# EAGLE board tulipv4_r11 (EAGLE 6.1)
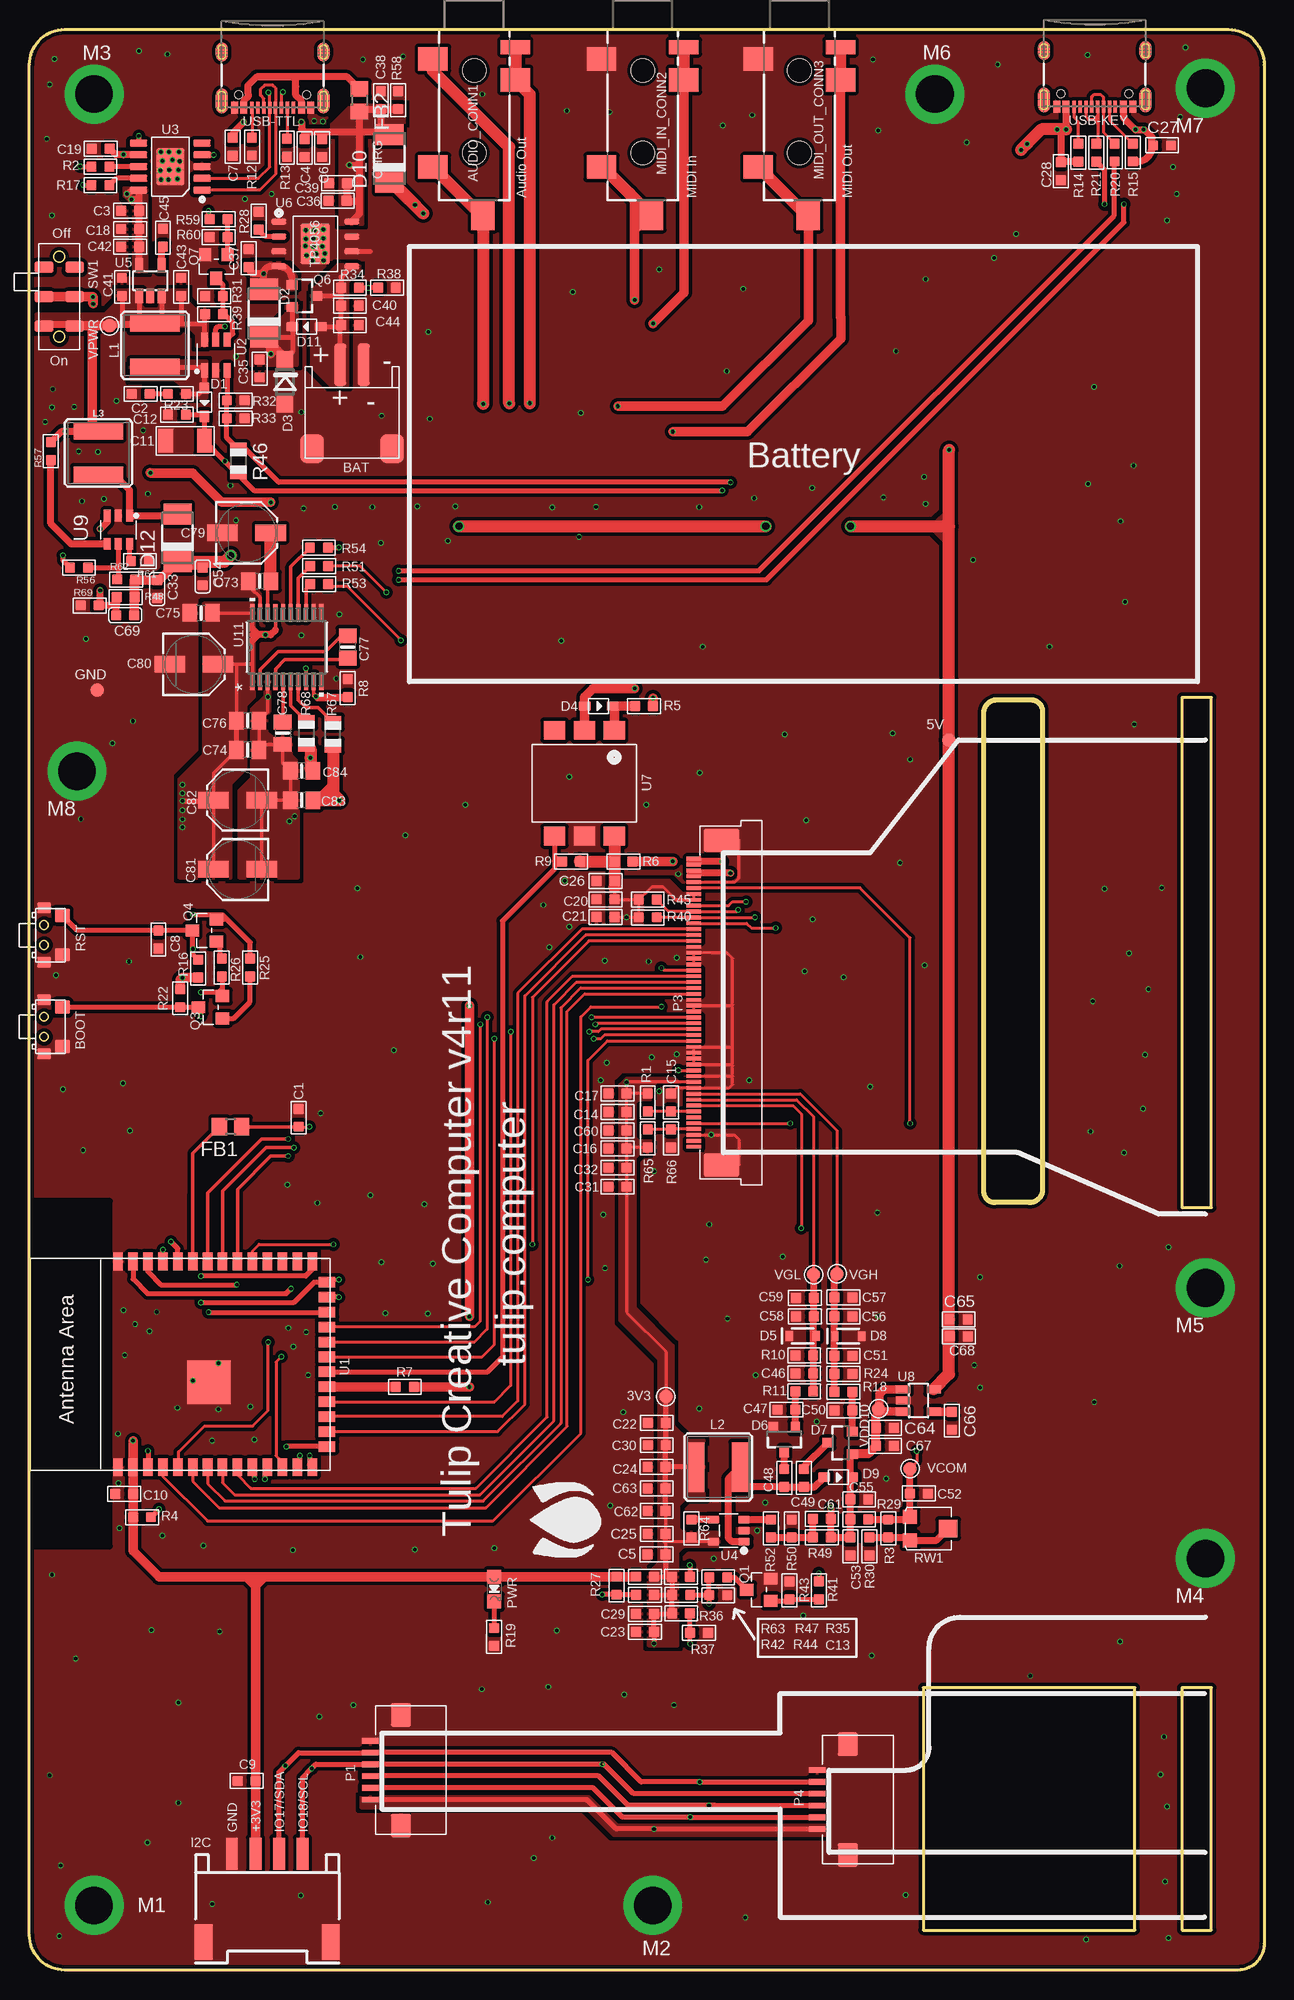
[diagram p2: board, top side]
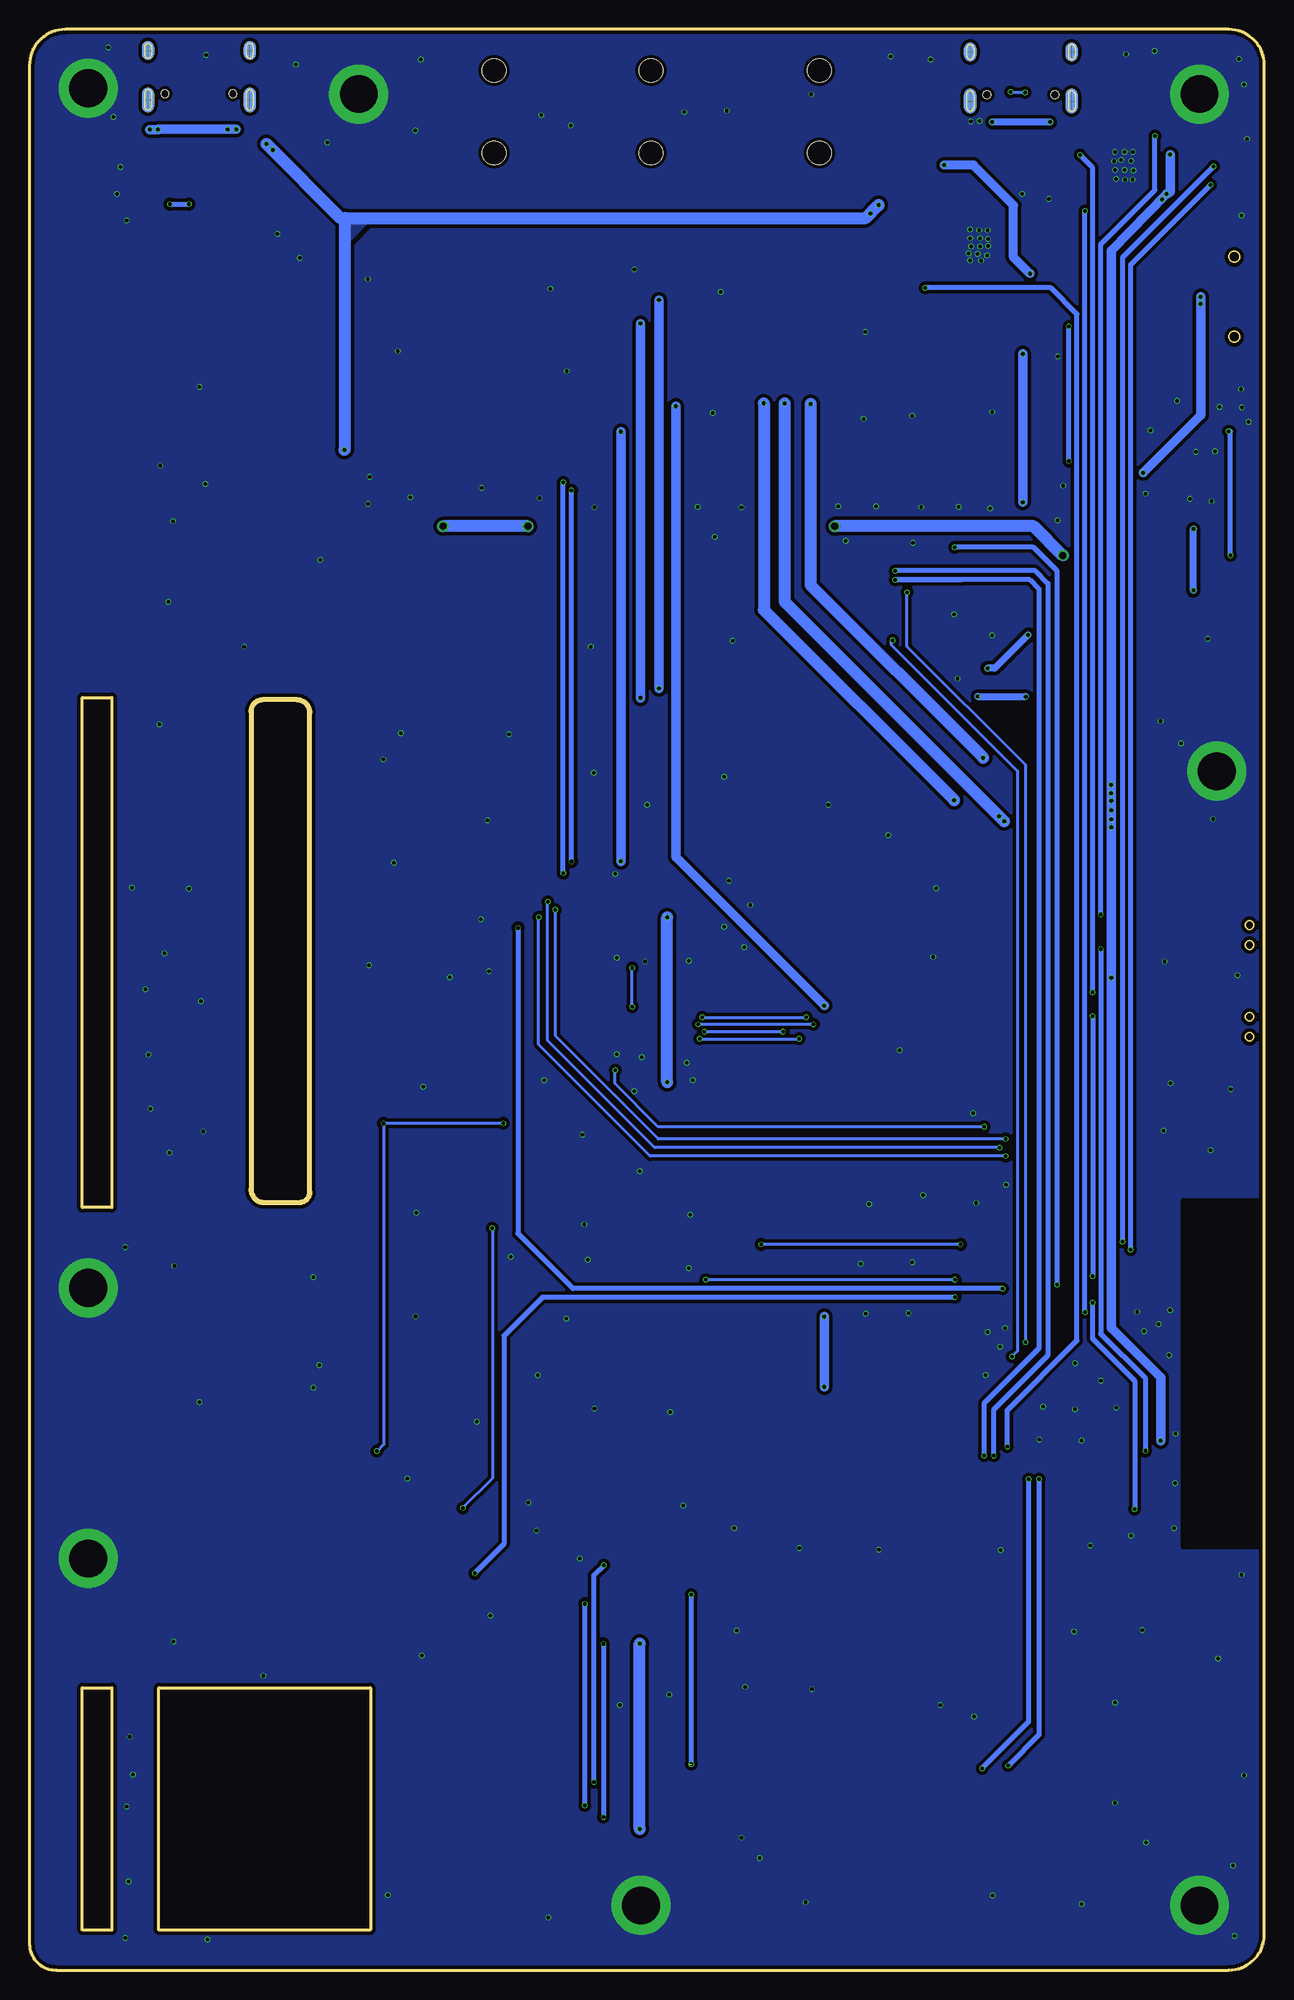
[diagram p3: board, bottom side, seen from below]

Size 105 x 165 mm. Coordinates in mm from the lower left corner, seen from the top.
Outline: 3,165 101.96,165 arc-90 105,161.96 105,2.26 arc-90 102.74,0 3,0 arc-90 0,3 0,162 arc-90 3,165
Outline: 85.03,65.25 82.09,65.25 arc-90 81.15,66.19 81.15,106.91 arc-90 82.25,108 85.17,108 arc-90 86.15,107.01 86.15,66.38 arc-90 85.03,65.25
Outline: 76,24 76,3.4 94,3.4 94,24 76,24
Outline: 98,108.2 98,64.82 100.5,64.82 100.5,108.2 98,108.2
Outline: 98,24 98,3.4 100.5,3.4 100.5,24 98,24
Copper layers (1*16): Top 0.035mm / dielectric 1.5mm / Bottom 0.035mm
Design rules: minimum track width 6mil, minimum drill 10mil, track to track 6mil, track to pad 6mil, pad to pad 6mil, via to via 6mil, smd to smd 0mil, copper to edge 10mil, drill to drill 10mil, minimum pad ring 3mil, minimum via ring 3mil, stop-mask expansion 2mil, vias tented up to drill 100mil, thermal gap 0mil
Net classes: 0 default: width 0.203 mm, drill 0.305 mm, clearance 0.152 mm; 1 vbat: width 0.254 mm, drill 0.305 mm, clearance 0.152 mm
tRestrict: area 0,36.1 to 6.8,65.4; area -3.4,136 to -2.6,142.5
bRestrict: area 0,36.1 to 6.8,65.4

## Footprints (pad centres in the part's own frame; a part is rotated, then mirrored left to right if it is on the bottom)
TP_4545 = smd 1.143 x 1.143: T 0,0
TP-D45MIL = smd 1.143 x 1.143: T 0,0
4UCONN_19269 = smd 2 x 2.5: 1 2.5,-3.5; 2 11.7,-3.5; 3 4.3,3.5 | smd 2.5 x 2: 4 15.8,0.75 | smd 1.2 x 2.5: 5 1.5,3.5 | hole 2: 3.5,0; 10.5,0
HW2-SMD-2.0-90D = smd 2 x 2.4: 3 3.4,-2.181; 4 -3.4,-2.181 | smd 1 x 3.6: + -1,4.953; - 1,4.953
2*4*3.5MM = smd 1.15 x 1.3: 1 -1.675,0; 2 1.675,0 | smd 0.9 x 1.2: 3 2.3,1.55; 4 -2.3,1.55
DISCRETE_C0603 = smd 0.889 x 0.889: 1 -0.762,0; 2 0.762,0
DISCRETE_C1206 = smd 1.27 x 2.032: 1 -1.651,0; 2 1.651,0
0603 = smd 0.889 x 0.889: 1 -0.762,0; 2 0.762,0
C0603 = smd 0.889 x 0.889: 1 0,0.762; 2 0,-0.762
0805-NO@1 = smd 1.24 x 1.5: 1 -0.95,0; 2 0.95,0
PANASONIC_C = smd 2.6 x 1.4: + 2.05,0; - -2.05,0
SOD323 = smd 1 x 0.8: + -1.2,0; - 1.2,0
DO-214AC = smd 1.8 x 2.4: A 2.025,0; C -2.025,0
SOD123 = smd 1.4 x 1.4: A 1.9,0; C -1.9,0
SOD-323 = smd 0.63 x 0.83: A 1.15,0; C -1.15,0
SOT23-3 = smd 0.8 x 0.9: 1 -0.95,-1; 2 0.95,-1; 3 0,1.1
R0805 = smd 1.3 x 1.5: 1 -0.95,0; 2 0.95,0
HW4-SMD-2.0-90D = smd 1.01 x 2.74: 1 -3,-0.1; 2 -1,-0.1; 3 1,-0.1; 4 3,-0.1 | smd 1.5 x 3: SS1 -5.4,7.4; SS2 5.4,7.4
CR54 = smd 4.2 x 1.4: P$1 0,1.85; P$2 0,-1.85
M2.5 = drill 3.2 pad 5: 1 0,0
1*6P-SMT1MM = smd 0.5 x 1.5: 1 -2.5,0; 2 -1.5,0; 3 -0.5,0; 4 0.5,0; 5 1.5,0; 6 2.5,0 | smd 2 x 1.7: 7 4.7,-2.6; 8 -4.7,-2.6
1*50P-SMT0.5MM = smd 0.3 x 1.3: 1 -12.25,0; 2 -11.75,0; 3 -11.25,0; 4 -10.75,0; 5 -10.25,0; 6 -9.75,0; 7 -9.25,0; 8 -8.75,0; 9 -8.25,0; 10 -7.75,0; 11 -7.25,0; 12 -6.75,0; 13 -6.25,0; 14 -5.75,0; 15 -5.25,0; 16 -4.75,0; 17 -4.25,0; 18 -3.75,0; 19 -3.25,0; 20 -2.75,0; 21 -2.25,0; 22 -1.75,0; 23 -1.25,0; 24 -0.75,0; 25 -0.25,0; 26 0.25,0; 27 0.75,0; 28 1.25,0; 29 1.75,0; 30 2.25,0; 31 2.75,0; 32 3.25,0; 33 3.75,0; 34 4.25,0; 35 4.75,0; 36 5.25,0; 37 5.75,0; 38 6.25,0; 39 6.75,0; 40 7.25,0; 41 7.75,0; 42 8.25,0; 43 8.75,0; 44 9.25,0; 45 9.75,0; 46 10.25,0; 47 10.75,0; 48 11.25,0; 49 11.75,0; 50 12.25,0 | smd 2 x 3: 51 13.79,-2.35; 52 -13.79,-2.35
CHIPLED_0805_NOOUTLINE = smd 1.2 x 1.2: A 0,-1.05; C 0,1.05
SOT23 = smd 1.016 x 1.143: 1 -0.95,-1.016; 2 0.95,-1.016; 3 0,1.016
DISCRETE_R0603 = smd 0.889 x 0.889: 1 -0.762,0; 2 0.762,0
R0603 = smd 0.889 x 0.889: 1 -0.762,0; 2 0.762,0
R0805' = smd 1.1 x 1.4: 1 -1,0; 2 1,0
TC33-3MM-SMD = smd 1.2 x 1.2: 1 -1,-1.625; 2 1,-1.625 | smd 1.5 x 1.6: 3 0,1.625
SMD-6-2.5MM = smd 1 x 1.6: 1 -2.5,1.3; 1@1 -2.5,-1.3; 2 0,1.3; 2@1 0,-1.3; 3 2.5,1.3; 3@1 2.5,-1.3
ESP32-­S2-­SOLO = smd 1.5 x 0.9: 1 -8.75,5.26; 2 -8.75,3.99; 3 -8.75,2.72; 4 -8.75,1.45; 5 -8.75,0.18; 6 -8.75,-1.09; 7 -8.75,-2.36; 8 -8.75,-3.63; 9 -8.75,-4.9; 10 -8.75,-6.17; 11 -8.75,-7.44; 12 -8.75,-8.71; 13 -8.75,-9.98; 14 -8.75,-11.25; 27 8.75,-11.25; 28 8.75,-9.98; 29 8.75,-8.71; 30 8.75,-7.44; 31 8.75,-6.17; 32 8.75,-4.9; 33 8.75,-3.63; 34 8.75,-2.36; 35 8.75,-1.09; 36 8.75,0.18; 37 8.75,1.45; 38 8.75,2.72; 39 8.75,3.99; 40 8.75,5.26 | smd 0.9 x 1.5: 15 -6.985,-12.5; 16 -5.715,-12.5; 17 -4.445,-12.5; 18 -3.175,-12.5; 19 -1.905,-12.5; 20 -0.635,-12.5; 21 0.635,-12.5; 22 1.905,-12.5; 23 3.175,-12.5; 24 4.445,-12.5; 25 5.715,-12.5; 26 6.985,-12.5 | smd 3.7 x 3.7: 41 -1.5,-2.46
SOT23-6 = smd 1.2 x 0.6: 1 -1.3,0.95; 2 -1.3,0; 3 -1.3,-0.95; 4 1.3,-0.95; 5 1.3,0; 6 1.3,0.95
ESOP-10-EP-150MIL = smd 1.5 x 0.6: 1 -2.7,2; 2 -2.7,1; 3 -2.7,0; 4 -2.7,-1; 5 -2.7,-2; 6 2.7,-2; 7 2.7,-1; 8 2.7,0; 9 2.7,1; 10 2.7,2 | smd 2.4 x 3.2: EP 0,0
SOT-23-5 = smd 0.7 x 1: 1 -0.95,-1.3; 2 0,-1.3; 3 0.95,-1.3; 4 0.95,1.3; 5 -0.95,1.3
SOT23-5 = smd 0.69 x 1.2: 1 -0.95,-1.3; 2 0,-1.3; 3 0.95,-1.3; 4 0.95,1.3; 5 -0.95,1.3
SOP8-1.27P = smd 1.27 x 0.51: 1 -3.1,1.905; 2 -3.1,0.635; 3 -3.1,-0.635; 4 -3.1,-1.905; 5 3.1,-1.905; 6 3.1,-0.635; 7 3.1,0.635; 8 3.1,1.905 | smd 2.5 x 3.4: 9 0,0
SOP-6-2.54MM = smd 1.6 x 1.8: 1 -4.5,2.54; 2 -4.5,0; 3 -4.5,-2.54; 4 4.5,-2.54; 5 4.5,0; 6 4.5,2.54
SOT-23-6 = smd 1 x 0.6: 1 -1.2,0.95; 2 -1.2,0; 3 -1.2,-0.95; 4 1.2,-0.95; 5 1.2,0; 6 1.2,0.95
PW20_TEX = smd 1.473 x 0.356: 1 -2.921,2.925; 2 -2.921,2.275; 3 -2.921,1.625; 4 -2.921,0.975; 5 -2.921,0.325; 6 -2.921,-0.325; 7 -2.921,-0.975; 8 -2.921,-1.625; 9 -2.921,-2.275; 10 -2.921,-2.925; 11 2.921,-2.925; 12 2.921,-2.275; 13 2.921,-1.625; 14 2.921,-0.975; 15 2.921,-0.325; 16 2.921,0.325; 17 2.921,0.975; 18 2.921,1.625; 19 2.921,2.275; 20 2.921,2.925
USB-C-16P-5 = smd 0.3 x 1: A5 -1.25,-0.34; A6 -0.25,-0.34; A7 0.25,-0.34; A8 1.25,-0.34; B5 1.75,-0.34; B6 0.75,-0.34; B7 -0.75,-0.34; B8 -1.75,-0.34 | smd 0.6 x 1: GND -3.225,-0.34; GND2 3.225,-0.34; VBUS1 -2.45,-0.34; VBUS2 2.45,-0.34 | smd 1 x 2.1: SHLD1 -4.32,-0.915; SHLD2 4.32,-0.915 | smd 1 x 2.1 bottom: SHLD3 -4.32,-0.915; SHLD4 4.32,-0.915 | smd 1 x 1.6: SHLD5 -4.32,-5.095; SHLD8 4.32,-5.095 | smd 1 x 1.6 bottom: SHLD6 -4.32,-5.095; SHLD7 4.32,-5.095 | hole 0.65: -2.89,-1.445; 2.89,-1.445

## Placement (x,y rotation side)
3V3  [TP_4545]  54.13,48.77 270 top
5V  [TP-D45MIL]  78.18,104.57 0 top
AUDIO_CONN1  19269  [4UCONN_19269]  37.82,165 270 top
BAT  JST-2P  [HW2-SMD-2.0-90D]  27.43,131.53 0 top
BOOT  TS24CA  [2*4*3.5MM]  2.8,80.2 90 top
C1  10pF/25V  [DISCRETE_C0603]  22.89,72.47 270 top
C2  10pF/50V  [DISCRETE_C0603]  9.47,134.01 0 top
C3  10uF  [DISCRETE_C0603]  8.56,149.58 0 top
C4  10uF  [DISCRETE_C0603]  23.39,154.91 90 top
C5  10uF  [DISCRETE_C0603]  53.31,35.36 0 top
C6  10uF  [DISCRETE_C0603]  24.89,154.91 90 top
C7  0.1uF  [DISCRETE_C0603]  17.3,155.02 90 top
C8  0.1uF  [DISCRETE_C0603]  10.97,87.63 270 top
C9  0.1uF  [DISCRETE_C0603]  18.47,16.08 180 top
C10  10uF  [DISCRETE_C0603]  8.05,40.49 180 top
C11  4.7uF/35V  [DISCRETE_C1206]  13.23,130.02 0 top
C12  0.1uF/50V  [DISCRETE_C0603]  12.55,132.23 0 top
C13  NC  [DISCRETE_C0603]  58.57,31.88 180 top
C14  0.1uF  [DISCRETE_C0603]  50.01,72.95 180 top
C15  100nF  [DISCRETE_C0603]  54.56,73.76 270 top
C16  10uF  [DISCRETE_C0603]  50.01,69.85 0 top
C17  0.1uF  [DISCRETE_C0603]  50.01,74.52 0 top
C18  0.1uF  [DISCRETE_C0603]  8.56,148.03 0 top
C19  0.1uF  [DISCRETE_C0603]  6.07,154.86 0 top
C20  10uF  [DISCRETE_C0603]  48.99,91.04 0 top
C21  0.1uF  [DISCRETE_C0603]  49,89.54 0 top
C22  10uF  [0603]  53.35,46.52 180 top
C23  10uF  [DISCRETE_C0603]  52.34,28.76 0 top
C24  0.1uF  [DISCRETE_C0603]  53.34,42.77 0 top
C25  0.1uF  [DISCRETE_C0603]  53.34,37.08 0 top
C26  0.1uF  [DISCRETE_C0603]  49,92.58 0 top
C27  10uF  [0603]  96.31,155.14 0 top
C28  0.1uF  [DISCRETE_C0603]  87.71,152.95 90 top
C29  10uF  [DISCRETE_C0603]  52.35,30.3 0 top
C30  0.1uF  [DISCRETE_C0603]  53.35,44.63 0 top
C31  10uF  [DISCRETE_C0603]  50.01,66.61 180 top
C32  0.1uF  [DISCRETE_C0603]  50.01,68.22 180 top
C33  22uF  [C0603]  10.87,117.42 0 top
C35  10uF  [0603]  19.58,136.17 90 top
C36  10uF  [0603]  26.21,150.44 0 top
C37  0.1uF  [0603]  18.63,145.55 90 top
C38  10uF  [0603]  29.88,158.99 90 top
C39  0.1uF  [0603]  26.25,151.93 180 top
C40  10uF  [0603]  27.25,141.5 0 top
C41  4.7uF/16V  [0603]  7.87,143.1 90 top
C42  10uF  [0603]  8.56,146.53 180 top
C43  10uF  [0603]  12.9,143.1 270 top
C44  0.1uF  [0603]  27.25,139.85 0 top
C45  NC  [0603]  11.35,147.29 90 top
C46  0.1uF  [DISCRETE_C0603]  65.89,50.72 0 top
C47  0.1uF  [DISCRETE_C0603]  64.36,47.65 0 top
C48  0.1uF  [DISCRETE_C0603]  64.19,41.83 90 top
C49  0.1uF  [DISCRETE_C0603]  65.86,41.83 270 top
C50  0.1uF  [DISCRETE_C0603]  69.22,47.57 0 top
C51  0.1uF  [DISCRETE_C0603]  69.22,52.22 180 top
C52  0.1uF  [DISCRETE_C0603]  75.64,40.51 180 top
C53  0.1uF  [DISCRETE_C0603]  69.8,36.02 90 top
C54  100nF  [C0603]  14.73,118.49 0 top
C55  0.1uF  [DISCRETE_C0603]  70.56,40.03 180 top
C56  1uF  [DISCRETE_C0603]  69.22,55.58 180 top
C57  1uF  [DISCRETE_C0603]  69.22,57.2 180 top
C58  1uF  [DISCRETE_C0603]  65.94,55.58 0 top
C59  1uF  [DISCRETE_C0603]  65.94,57.15 0 top
C60  100nF  [DISCRETE_C0603]  50.01,71.37 0 top
C61  10pF/25V  [DISCRETE_C0603]  67.39,38.35 0 top
C62  0.1uF  [DISCRETE_C0603]  53.34,39.04 0 top
C63  10uF  [DISCRETE_C0603]  53.34,40.97 0 top
C64  4.7uF/16V  [0603]  72.76,44.57 0 top
C65  10uF  [0603]  79.01,55.32 0 top
C66  NC  [0603]  78.46,46.71 270 top
C67  0.1uF/16V  [DISCRETE_C0603]  72.76,46.1 180 top
C68  0.1uF  [DISCRETE_C0603]  79.03,53.87 180 top
C69  22pF  [C0603]  8.15,115.19 270 top
C73  0.1uF  [0805-NO@1]  19.58,118.08 180 top
C74  0.1uF  [0805-NO@1]  18.57,103.73 180 top
C75  0.1uF  [0805-NO@1]  14.6,115.39 0 top
C76  0.1uF  [0805-NO@1]  18.57,106.22 180 top
C77  2.2uF  [0805-NO@1]  27.08,112.5 90 top
C78  2.2uF  [0805-NO@1]  21.54,105.16 270 top
C79  10uF  [PANASONIC_C]  18.47,122.2 0 top
C80  10uF  [PANASONIC_C]  14,111.02 0 top
C81  10uF  [PANASONIC_C]  17.7,93.57 180 top
C82  10uF  [PANASONIC_C]  17.7,99.47 180 top
C83  2.2nF  [0805-NO@1]  23.16,99.47 180 top
C84  2.2nF  [0805-NO@1]  23.16,101.96 180 top
D1  1N4148WS  [SOD323]  14.88,133.3 270 top
D2  SS54  [DO-214AC]  19.96,140.87 90 top
D3  W8/5.1V  [SOD123]  21.72,135.03 270 top
D4  1N4148WS  [SOD323]  48.41,107.47 0 top
D5  7.5V  [SOD-323]  65.76,53.92 0 top
D6  200mA/70V  [SOT23-3]  64.19,45.16 180 top
D7  200mA/70V  [SOT23-3]  68.99,44.83 90 top
D8  16V  [SOD-323]  69.62,53.9 0 top
D9  1N4148WS  [SOD323]  68.78,41.91 0 top
D10  SS54  [DO-214AC]  30.62,154.02 90 top
D11  B5819WS  [SOD323]  23.57,139.73 180 top
D12  SS54  [DO-214AC]  12.6,121.77 90 top
FB1  100Mhz@120R  [R0805]  17.1,71.7 180 top
FB2  100Mhz@120R  [R0805]  28.06,158.98 270 top
GND  [TP-D45MIL]  5.77,108.81 0 top
I2C  [HW4-SMD-2.0-90D]  20.22,9.79 180 top
L1  10µH/±30%  [CR54]  10.67,138.15 0 top
L2  10µH/±30%  [CR54]  58.57,42.77 90 top
L3  3.3µH/±30%/3.4A  [CR54]  5.87,128.98 0 top
M1  M2.5  [M2.5]  5.5,5.5 0 top
M2  M2.5  [M2.5]  53,5.5 0 top
M3  M2.5  [M2.5]  5.5,159.5 0 top
M4  M2.5  [M2.5]  100,35 0 top
M5  M2.5  [M2.5]  100,58 0 top
M6  M2.5  [M2.5]  77,159.5 0 top
M7  M2.5  [M2.5]  100,160 0 top
M8  M2.5  [M2.5]  4.04,101.93 0 top
MIDI_IN_CONN2  19269  [4UCONN_19269]  52.15,165 270 top
MIDI_OUT_CONN3  19269  [4UCONN_19269]  65.48,165 270 top
P1  1X6P-1MM  [1*6P-SMT1MM]  29,17 90 top
P3  150P-0.5MM  [1*50P-SMT0.5MM]  56.5,82.25 90 top
P4  1X6P-1MM  [1*6P-SMT1MM]  67,14.5 90 top
PWR  NC  [CHIPLED_0805_NOOUTLINE]  39.52,32.4 180 top
Q1  S8050  [SOT23]  62.03,32.33 90 top
Q3  S8050  [SOT23]  15.41,81.86 90 top
Q4  S8050  [SOT23]  14.88,88.39 90 top
Q6  MOSFET-PCHANNEL  [SOT23-3]  23.34,142.34 270 top
Q7  S8050  [SOT23]  15.9,144.83 180 top
R1  10K  [DISCRETE_R0603]  52.58,73.76 90 top
R2  0R  [R0603]  6.05,153.34 0 top
R3  3.48K  [DISCRETE_R0603]  73.03,37.54 90 top
R4  NC  [R0603]  9.58,38.51 0 top
R5  220R  [R0603]  52.27,107.47 0 top
R6  33R  [R0603]  50.52,94.26 0 top
R7  10R  [R0603]  31.93,49.58 0 top
R8  0R  [DISCRETE_R0603]  27.08,108.99 90 top
R9  470R  [R0603]  46.05,94.26 180 top
R10  4.3K  [DISCRETE_R0603]  65.89,52.27 0 top
R11  2K  [DISCRETE_R0603]  65.89,49.2 0 top
R12  5.1K  [DISCRETE_R0603]  18.92,155.04 90 top
R13  5.1K  [DISCRETE_R0603]  21.89,154.94 90 top
R14  56K  [DISCRETE_R0603]  89.2,154.51 90 top
R15  56K  [DISCRETE_R0603]  93.83,154.53 90 top
R16  10K  [R0603]  14.35,85.14 270 top
R17  0R  [R0603]  6.05,151.76 0 top
R18  1.2K  [DISCRETE_R0603]  69.22,49.15 0 top
R19  NC  [DISCRETE_R0603]  39.52,28.32 90 top
R20  51R  [R0603]  92.28,154.53 270 top
R21  51R  [R0603]  90.73,154.51 270 top
R22  10K  [R0603]  12.83,82.63 90 top
R23  50R  [DISCRETE_R0603]  12.55,134.01 0 top
R24  4.3K  [DISCRETE_R0603]  69.22,50.7 180 top
R25  10K  [R0603]  18.77,85.24 90 top
R26  10K  [R0603]  16.37,85.24 270 top
R27  NC  [R0603]  49.91,32.69 90 top
R28  1.2K  [R0603]  19.48,148.74 90 top
R29  10KR  [DISCRETE_R0603]  70.56,38.33 180 top
R30  2K  [DISCRETE_R0603]  71.42,36.02 90 top
R31  NC  [DISCRETE_R0603]  15.7,142.32 0 top
R32  3.6R  [DISCRETE_R0603]  17.55,133.45 180 top
R33  3.6R  [DISCRETE_R0603]  17.55,131.93 180 top
R34  470K  [R0603]  27.25,143.03 180 top
R35  0R  [R0603]  58.57,33.4 180 top
R36  NC  [DISCRETE_R0603]  55.42,30.33 180 top
R37  NC  [DISCRETE_R0603]  56.95,28.68 0 top
R38  470K  [R0603]  30.4,143.03 180 top
R39  10K  [DISCRETE_R0603]  15.7,140.79 180 top
R40  10K  [DISCRETE_R0603]  52.58,89.51 180 top
R41  4.7K  [DISCRETE_R0603]  67.13,32.28 90 top
R42  5.1K  [DISCRETE_R0603]  52.35,31.91 0 top
R43  10K  [DISCRETE_R0603]  64.64,32.28 270 top
R44  10K  [DISCRETE_R0603]  55.43,31.9 180 top
R45  10K  [DISCRETE_R0603]  52.58,91.01 180 top
R46  470  [R0805']  17.79,128.31 90 top
R47  5.1K  [DISCRETE_R0603]  55.41,33.43 180 top
R48  88.7K  [DISCRETE_R0603]  8.18,116.74 0 top
R49  100K  [DISCRETE_R0603]  67.39,36.78 0 top
R50  13K  [DISCRETE_R0603]  64.82,37.54 270 top
R51  0R  [R0603]  24.64,119.35 180 top
R52  100K  [DISCRETE_R0603]  63.07,37.54 90 top
R53  0R  [R0603]  24.64,117.83 180 top
R54  0R  [R0603]  24.61,120.95 180 top
R56  NC  [DISCRETE_R0603]  4.22,119.25 180 top
R57  100K  [DISCRETE_R0603]  1.83,129.13 90 top
R58  100k  [R0603]  31.34,158.99 90 top
R59  4.7K  [DISCRETE_R0603]  16.1,148.87 180 top
R60  10K  [DISCRETE_R0603]  16.1,147.35 0 top
R61  NC  [DISCRETE_R0603]  9.4,119.79 180 top
R62  0R  [DISCRETE_R0603]  8.23,118.24 0 top
R63  0R  [R0603]  52.35,33.45 0 top
R64  4.3K  [DISCRETE_R0603]  56.29,37.54 270 top
R65  10K  [DISCRETE_R0603]  52.58,70.71 270 top
R66  NC  [DISCRETE_R0603]  54.56,70.71 90 top
R67  470  [R0805']  25.81,105.08 90 top
R68  470  [R0805']  23.57,105.16 90 top
R69  12K  [DISCRETE_R0603]  5.13,116.03 0 top
RST  TS24CA  [2*4*3.5MM]  2.8,88 90 top
RW1  TC33X-2-103E  [TC33-3MM-SMD]  76.5,37.54 270 top
SW1  JS102011JAQN  [SMD-6-2.5MM]  2.54,142.27 270 top
U1  ESP32­S2­SOLO  [ESP32-­S2-­SOLO]  12.8,51.5 90 top
U2  RY3730  [SOT23-6]  15.85,137.31 90 top
U3  CH340K  [ESOP-10-EP-150MIL]  11.99,153.34 180 top
U4  SGM6601YTN5G/TR  [SOT-23-5]  59.46,37.36 90 top
U5  SPX3819  [SOT23-5]  10.29,143.64 0 top
U6  TP4056  [SOP8-1.27P]  24.31,146.76 0 top
U7  H11L1SR2M  [SOP-6-2.54MM]  47.19,100.91 270 top
U8  SPX3819  [SOT23-5]  75.6,48.43 270 top
U9  HX3608  [SOT-23-6]  7.57,122.45 270 top
U11  U11  [PW20_TEX]  21.89,112.47 90 top
USB-KEY  [USB-C-16P-5]  90.58,158.1 180 top
USB-TTL  [USB-C-16P-5]  20.69,157.99 180 top
VCOM  [TP_4545]  74.88,42.62 0 top
VDD10  [TP_4545]  72.21,47.72 0 top
VGH  [TP_4545]  68.68,59.21 0 top
VGL  [TP_4545]  66.67,59.13 90 top
VPWR  [TP_4545]  6.81,139.8 0 top

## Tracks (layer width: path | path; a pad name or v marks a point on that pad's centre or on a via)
3.3V  (via drill 0.3)
  Top 0.254: C16.2 C60.2 C14.1 C17.2 | R65.2 50.77,69.95 C16.2 | R1.2 C17.2 | C17.2 v50.77,75.5 P3.12 | R45.2 52.91,92.1 53.9,92.1 55,91 P3.43 P3.44 | R45.2 R40.2 51.79,89.54 C21.2 | C20.2 51.79,91.04 R45.2 | C16.2 C32.1 C31.1 50.78,55.93 54.11,52.59 C22.1 54.08,46.49 54.08,36.41 | 54.08,36.41 C5.2 | U4.5 56.31,36.41 | 56.31,36.41 54.08,36.41 | R64.2 56.31,36.78 56.31,36.41 | R6.1 49.76,95.68 49.73,95.71
  Top 0.305: C20.2 49.76,92.05 C26.2
  Top 0.406: P4.1 v53.11,12 49.9,12 47.4,14.5 P1.1 | R44.2 R36.2 54.63,30.3 C29.2 C23.2 v53.11,27.77 v53.11,27.76 | R42.2 54.65,31.91 R44.2 | R44.2 54.66,33.41 R47.2 54.62,33.45 54.05,33.45 | R63.2 54.05,33.45 | C5.2 54.08,33.48 54.05,33.45 | L2.P$1 C24.2 | 54.08,36.41 54.08,37.06 C25.2 | C62.2 C63.2 C24.2 | C24.2 C30.2 C22.1 54.11,48.75 3V3.T
  Top 1.016: R9.1 R6.1 | U7.6 49.73,95.71 49.73,92.07 49.76,92.05
  Bottom 1.016: v50.77,75.5 v50.77,89.5 | v53.11,12 v53.11,27.76
  pour Top: 28.22,14.76 47.6,14.76 50.01,12.34 67.74,12.34 67.74,11.43 49.68,11.43 47.35,13.77 28.22,13.77
  pour Top: 52.65,27.53 52.65,33.78 53.54,34.67 53.54,51.87 50.22,55.19 50.22,75.31 50.77,75.87 54.71,75.87 55.35,75.46 55.32,75.46 53.26,75.41 52.88,75.03 52.88,73.99 51.79,73.99 51.49,73.69 51.49,70.84 51.79,70.54 52.86,70.54 52.86,69.44 51.92,69.44 51.49,69.01 51.49,56.36 54.74,53.11 54.74,46.35 56.03,45.06 57.38,45.06 57.38,40.08 55.8,40.08 55.19,39.47 55.19,37.59 55.52,37.26 58.62,37.26 58.62,35.97 55.63,35.97 55.12,35.46 55.12,27.53
  pour Top: 49.35,89 52.2,89 52.2,91.29 52.78,91.87 53.98,91.87 54.89,90.96 57,90.96 57,91.54 55.58,91.54 54.48,92.63 50.04,92.63 49.35,91.95
5V  (via drill 0.3, 0.6)
  Top 0.254: 33.5,149.34 v33.48,149.34 arc-90 v33.48,149.35 | v33.48,149.35 arc90 v33.48,149.35
  Top 0.406: C28.2 87.72,153.73 87.72,153.74 | D10.C 30.59,152 30.59,151.84
  Top 0.584: v88.13,156.5 v88.14,156.5 | v88.14,156.5 arc90 v88.14,156.5
  Top 0.61: USB-KEY.VBUS1 93.03,157.49 94.06,156.46 94.11,156.46 | USB-KEY.VBUS2 88.13,157.08 v88.14,156.5 | 94.11,156.46 94.82,156.46 95.38,155.91 arc-90 95.38,155.9 95.38,155.88 arc-90 95.45,155.81 95.45,155.68 | v94.06,156.49 94.08,156.49 94.11,156.46 | R15.1 94.22,153.77 arc90 95.45,155 95.45,155.68 | R14.1 87.7,153.75 arc90 87.69,153.74 87.72,153.74 arc90 87.74,153.76 87.74,156.11 arc-90 v88.13,156.5 | C27.1 95.45,155.68 | 8.94,118.19 C33.1 10.87,118.16 10.95,118.16 12.17,119.38 14.61,119.38 C54.1 | 5V.T 78.23,104.57 78.23,104.64 78.2,104.67
  Top 0.711: 78.25,53.87 C68.2 78.25,53.87 | 78.25,53.87 78.21,53.91 78.16,53.91 78.09,53.84 | 78.25,53.87 78.2,53.83 | C65.1 78.2,55.28
  Top 0.813: C69.1 8.91,118.16 | 8.91,118.16 8.94,118.19 | 8.91,118.16 10.87,118.16 11.02,118.16 D12.C | R48.2 8.94,118.19 | 8.94,118.19 R62.2
  Top 1.016: v88.14,156.5 86.07,156.5 v84.84,155.27 v84.32,154.75 v84.31,154.75 | v32.8,150.08 31.04,151.84 31.01,151.84 | 31.01,151.84 30.59,151.84 30.28,151.84 | 30.46,151.65 31.2,151.65 | 31.2,151.65 33.5,149.34 | 31.2,151.65 31.01,151.84 | U8.5 78.2,50.68 78.2,53.83 78.2,55.28 78.2,104.67 78.2,122.73 | 78.2,122.73 v78.2,129.26 | D12.C 16.59,119.74 v17.12,120.27 | v36.52,122.76 v62.61,122.76 | v69.83,122.76 78.03,122.76 arc-90 78.05,122.73 78.2,122.73
  Bottom 0.584: v87.4,156.5 arc90 v87.39,156.49 | v94.06,156.48 arc-90 v94.06,156.49
  Bottom 0.61: 94.05,156.5 v94.06,156.49
  Bottom 0.813: 94.05,156.5 v88.14,156.5 v87.4,156.5 | v94.76,156.48 v94.06,156.48
  Bottom 1.016: 78.53,148.96 v84.84,155.27 | 78.53,148.96 78.16,148.96 | 78.16,148.96 33.88,148.96 32.8,150.04 v32.8,150.08 | v78.2,129.26 78.16,129.3 78.16,148.96 | 78.53,148.96 78.49,148.93 78.05,148.93 78.08,148.96 78.14,148.96 78.14,148.91 | v17.12,120.27 19.61,122.76 v36.52,122.76 | v62.61,122.76 v69.83,122.76
  pour Bottom: 75.98,148.82 77.87,146.93 78.54,146.93 78.43,147.59 78.49,149.27 75.98,149.27
  pour Top: 78,124.1 76.83,122.94 76.83,122.38 77.83,121.39 78.05,121.39 78.05,124.13 78.03,124.13
+3V3  (via drill 0.3)
  Top 0.305: 18.97,113.56 U11.20 C75.2 | 18.97,113.56 18.97,110.9 | U11.1 | U11.17 20.92,113.94 | 19,113.54 18.97,113.56 | C80.+ 17.7,111.02 | 17.7,111.02 18.84,111.02 18.97,110.9 | C76.2 17.62,110.94 17.7,111.02 | C74.2 15.65,101.77 C82.+ C81.+ | U11.8 v23.52,110.69 | v23.52,110.69 | U11.1 18.97,110.9 | 18.97,110.9
  Top 0.406: 8.02,154.34 v8,154.36 | C74.2 C76.2 | v13,99.4 15.59,99.4 C82.+
  Top 0.61: 20.92,113.94 20.52,113.54 v20.06,113.54 19.43,113.54 | 19.43,113.54 19,113.54 | U3.7 8.02,154.34 7.36,154.34 C19.2 | v8.31,151 8.74,151.34 U3.10 9.32,151.31 9.32,150.44 | 18.85,114.22 18.85,114.12 19.43,113.54 | 19.43,113.54 18.82,112.93 | U5.5 9.34,146.52 C42.1 C18.2 C3.2 9.32,150.44 | v8.69,150.55 9.22,150.55 9.32,150.44
  Top 0.813: 19.48,33.45 11.04,33.45 11.02,33.43 8.81,35.64 R4.1 C10.1 U1.2 v8.81,45 | 19.48,33.45 PWR.A R27.2 R63.1 | I2C.3 C9.1 19.23,32.69 | 19.23,32.69 19.23,33.19 19.48,33.45 | R22.2 12.83,84.21 v13,84.38 R16.2 | 19.23,32.69 19.99,33.45 | 19.23,32.69 19.18,32.69 18.47,33.4
  Bottom 0.61: v20.06,113.54 22.91,110.69 v23.52,110.69
  Bottom 0.813: v8.81,45 8.81,50.39 13,54.58 v13,84.38 v13,99.4 13,146.21 v8.31,151 8,151.21 v8,154.36
  other vias: 13.03,100.77 13,97.83 13.03,100.06 13,98.61 13,97.16
  pour Top: 15.44,116.26 19.1,116.26 19.1,108.18 18.39,107.47 18.39,102.08 17.12,100.81 17.12,92.81 12.75,92.81 12.75,101.3 14.83,103.38 14.83,116.26
  pour Top: 8.86,144.35 8.86,149.99 8.05,150.8 8.05,151.56 9.96,151.56 9.96,144.4 9.96,144.35
AGND  (via drill 0.3)  (1 unrouted)
  Top 0.254: R8.1 24.49,108.23 24.17,108.55 U11.9 24.17,108.29 v24.35,108.28
  Top 0.305: C81.- C82.- C83.2 C84.2 21.54,102.63 C78.2 19.63,104.21 19.52,104.32 | C74.1 19.52,104.32 | 19.52,104.32 C76.1 20.27,106.97 v20.27,108.25 U11.3 | 24.18,108.84 24.18,108.31 24.49,108 27.15,108 27.15,108.43 27.03,108.43 26.95,108.36 24.41,108.36 24.23,108.53
  Top 0.406: AUDIO_CONN1.1 34.32,161.97
  Top 1.016: v40.79,133.2 40.79,154.99 34.32,161.46 AUDIO_CONN1.1
  Bottom 0.254: 20.3,108.28 v20.27,108.25
  Bottom 0.61: v24.35,108.28 20.3,108.28
  Bottom 1.016: v40.79,133.2 40.79,116.36 v22.1,97.66
  other vias: 22.56,98.09
  pour Top: 17.86,92.81 17.86,100.33 18.9,101.37 18.9,107.24 20.04,108.38 20.04,110.29 20.42,110.29 20.42,106.96 20.19,106.73 20.19,105.31 20.6,104.9 22.28,104.9 22.28,103.33 22.83,102.77 22.83,92.89 22.83,92.81
AVDD10  (via drill 0.3)
  Top 0.254: P3.8 64.93,73.5 65.63,72.8 v65.63,63.07
  Top 0.61: v68.15,39.29 C61.2 R49.2 C53.2 R29.2 C55.2 69.8,41.96 | 69.8,41.96 69.8,43.69 D7.1 | D9.- 69.85,41.91 69.8,41.96
  Top 0.711: U8.3 72.42,47.48 72.29,47.61 72.29,47.78 | U8.1 72.66,49.38 72.29,49 72.29,47.78 | VDD10.T 72.21,47.78 72.18,47.81 72.27,47.81 72.29,47.78
  Top 0.762: C64.1 71.32,43.89 70,43.89 D7.1 | C64.1 | C64.1 C67.2 72,47.06 72.42,47.48
  Bottom 0.254: v65.63,63.07 65.63,41.81 v68.15,39.29
BCLK
  Top 0.305: U11.13 23.52,117.47 R53.2
D+
  Top 0.254: U3.1 19.58,151.33 20.94,152.69 USB-TTL.A6 20.94,160.04 20.7,160.27 19.99,160.27 19.66,159.94 19.66,159.38 19.94,159.11 USB-TTL.B6
D-  (via drill 0.3)
  Top 0.254: U3.2 19.47,152.34 20.44,153.31 USB-TTL.A7 20.44,159.52 v20.32,159.64 | USB-TTL.B7 21.44,159.54 v21.57,159.66
  Bottom 0.254: v21.57,159.66 v20.32,159.64
DCLK  (via drill 0.3)
  Top 0.254: C1.2 v23.8,71.7 | 56.33,76.5 P3.14 v55.2,76.5 v55.19,76.5
  Top 0.305: FB1.1 | FB1.1 C1.2
  Bottom 0.254: v23.8,71.7 51.54,71.7 55.19,75.36 v55.19,76.5
DIN
  Top 0.305: U11.14 22.87,118.35 R51.2
DTR  (via drill 0.3)
  Top 0.406: U3.4 v15.66,154.34 v15.67,154.33 | Q3.2 16.42,83.44 | 16.42,83.44 16.42,84.42 R26.2 | v14.58,83.14 16.13,83.14 16.42,83.44
  Bottom 0.406: v14.58,83.14 14.58,153.24 v15.67,154.33
ENABLE
  Top 0.61: U9.4 3.56,121.26 1.83,122.99 R57.1
GND  (via drill 0.3)
  Top 0.254: P3.51 60.35,96.04 60.35,92.86 59.99,92.5 P3.46 | v57.96,71.02 56.14,71 P3.3 59.96,71 60.35,70.61 60.35,68.46 P3.52 | 59.79,76 59.79,75.29 59.51,75 P3.11 55.04,75 C15.1 | 59.79,76 59.79,76.91 | 59.79,76.91 59.79,82.07 | 59.79,82.07 59.79,86.03 59.33,86.49 58.01,86.49 P3.34 P3.32 | P3.13 59.79,76 | 59.79,76.91 59.7,77 P3.15 P3.18 59.73,78.5 59.74,78.51 | 59.79,82.07 59.72,82 P3.25 P3.24
  Top 0.305: U11.19 19.62,116.73 18.87,117.47 18.87,117.85 C73.2
  Top 0.406: U6.6 29.01,146.13
  other vias: 96.47,19.84 96.57,7.54 74.9,102.93 69.24,84.4 45.52,92.61 91.44,91.95 71.51,75.11 93.95,105.92 46.2,142.67 1.73,16.56 90.22,71.3 94.87,77.83 66.6,89.36 96.19,16.64 15.54,5.61 96.29,92.02 52.93,77.62 22.4,35.71 94.69,73.23 96.85,2.72 8.99,54.91 66.04,97.76 42.9,9.53 10.03,10.85 24.66,21.54 12.67,14.22 96.72,13.92 23.14,132.46 44.45,11.25 59.31,135.94 80.85,49.53 2.54,2.9 76.12,85.44 37.06,99.06 23.09,6.32 43.71,90.55 2.67,8.89 85.12,25.02 90.42,82.37 38.99,5.77 95.15,83.39 89.87,2.59 90.02,126.36 86.74,112.52 46.74,121.87 96.85,61.47 1.93,33.6 12.67,22.73 7.95,75.41 2.84,74.9 11.33,36.93 10.36,28.91 14.78,36.09 3.94,26.49 2.26,84.58 8.46,85.75 8.56,71.37 39.52,35.89 7.54,45.59 8,56.11 8.1,52.3 10.82,55.96 33.88,55.8 22.02,54.59 16.08,51.61 13.89,50.11 22.45,53 18.8,47.89 23.7,50.6 10.21,54.33 12.57,47.8 19.12,45.1 15.54,45.03 16.08,47.68 30.25,55.85 24.49,65.23 4.8,113.18 16.18,28.78 60.71,142.95 57.53,60.4 8.81,106.2 31.98,96.49 4.57,69.7 24.77,72.85 21.94,66.77 34.32,60.05 29.01,65.89 33.58,65.13 30.99,78.21 27.89,91.97 28.14,86.13 45.92,88.7 4.37,97.87 46.89,132.41 92.74,27.94 90.55,48.29 33.91,139.27 93.17,116.33 7.06,104.29 93.88,127.91 92.79,123.19 92.68,59.87 29.87,121.34 45.21,113 93.09,69.49 44.22,86.97 93.52,86.46 2.13,162.48 1.47,155.7 9.32,163.17 11.73,162.89 1.73,160.32 31.78,162.69 38.51,159.49 28.37,162.43 45.69,158.09 71.73,162.46 58.95,156.84 61.47,157.71 82.35,162.03 98.3,163.47 97.87,157.56 89.97,162.84 97.26,153.31 97.56,151 96.72,148.77 79.68,155.4 82.02,145.57 49.33,157.96 73.69,137.64 83.9,147.62 1.93,149.17 64.21,105.05 90.53,134.62 57.25,112.52 73.41,105.16 61.21,75.67 65.91,84.91 80.85,58.93 48.59,75.67 53.57,74.73 44.86,28.88 44.12,24.08 27.53,22.53 38.46,23.88 32.77,35.76 50.5,47.45 49.4,39.5 45.06,37.57 56.95,47.73 48.79,64.24 48.95,59.69 53.11,67.92 57.81,63.4 59.36,55.4 61.77,50.6 66.95,46.63 72.11,64.39 72.16,55.58 80.35,51.44 65.81,30.15 71.63,26.75 74.52,6.38 60.88,4.47 50.6,23.42 54.81,22.53 76.23,143.76 72.19,156.41 48.92,85.8 52.65,85.75 55.04,86.06 55.04,77.88 49.1,77.14 23.53,54.23 29.92,60.17 23.52,147.93 24.23,147.93 24.99,147.98 24.99,147.24 24.16,147.24 23.5,147.19 23.47,146.58 24.16,146.56 24.92,146.56 25.12,145.95 24.38,145.9 23.57,145.77 24.08,145.34 25.02,145.36 20.59,151 18.31,150.57 11.18,154.58 11.86,154.58 12.7,154.58 12.78,153.8 12.17,153.9 11.33,153.82 11.13,153.01 11.89,153.03 12.67,153.06 12.6,152.3 11.84,152.22 11.2,152.22 26.37,115.27 23.14,113.49 26.09,109.8 17.58,123.27 17.55,137.19 34.06,131.9 35.59,121.51 45.92,101.45 52.45,99.09 57,101.8 55.17,93.19 74.03,94.13 64.06,60.66 80.26,119.89 7.42,133.43 1.98,134.42 29.95,132.16 23.32,124.28 61.87,37.36 58.19,34.98 62.56,39.75 72.85,41.78 7.67,37.59 7.57,41.4 53.54,144.6 17.09,126.21 24.21,157.23 24.94,157.17 25.98,124.41 29.16,124.38 32.99,124.46 36.22,124.43 44.45,124.36 48.18,124.41 56.95,124.38 61.62,125.15 66.55,126.01 72.62,125.22 76.07,126.95 76.2,124.66 4.47,124.89 6.32,125.07 10.08,125.53 4.19,129.11 5.82,129.08 3.81,132.92 1.91,132.87 1.35,131.62 9.68,130.91
  pour Top (isolate 0.305, rank 6): -10,180 -10,-20 150,-20 150,180
  pour Bottom (isolate 0.305, rank 6): -5,-20 150,-20 150,180 -5,180
IO0  (via drill 0.3)
  Top 0.406: U1.27 24.05,59.56 23.5,59 v14.58,59 | BOOT.2 12.82,81.88 R22.1 Q3.3 | Q3.3 | Q3.3 14.58,81.67 v14.58,81.11
  Bottom 0.406: v14.58,81.11 v14.58,59
IO1  (via drill 0.3)
  Top 0.254: P3.39 60.99,89 61.38,88.6 v63.45,88.6
  Top 0.406: U1.39 8.81,58.75 10.03,57.53 21.85,57.53 v22.26,57.94
  Bottom 0.406: v63.45,88.6 63.45,62.61 58.78,57.94 v22.26,57.94
IO2  (via drill 0.3)
  Top 0.406: U1.38 10.08,59.36 11.18,58.27 v17.63,58.27 | R54.1 v26.31,120.95
  Bottom 0.406: v17.63,58.27 17.63,118.97 19.63,120.98 26.29,120.98 v26.31,120.95
IO3  (via drill 0.3)
  Top 0.406: R38.2 v28.83,143.03 R34.1 | U1.15 21.86,44.52 v21.84,44.5
  Bottom 0.406: v21.84,44.5 21.84,47.6 15.93,53.52 15.93,140.79 18.16,143.03 v28.83,143.03
IO4  (via drill 0.3)
  Top 0.254: U1.4 11.35,41.97 15.14,38.18 39.42,38.18 46.89,45.64 46.89,81.05 47.74,81.9 v53.75,81.9 | P3.31 53.95,85 v53.75,85.2
  Bottom 0.254: v53.75,81.9 v53.75,85.2
IO5  (via drill 0.3)
  Top 0.254: U1.5 12.69,42.75 12.69,44.06 14.9,46.27 18.99,46.27 20.3,47.58 v20.3,53.4 | v30.37,117.14 28.14,119.36 R51.1 | R51.1 | R51.1
  Bottom 0.254: v20.3,53.4 20.3,102.48 20.31,102.47 20.31,102.48 30.37,112.54 v30.37,117.14
IO6
  Top 0.254: U1.6 13.89,41.56 16.13,39.32 38.81,39.32 45.72,46.23 45.72,81.51 47.21,83 P3.27
IO7
  Top 0.254: U1.7 15.16,41.35 16.64,39.88 38.58,39.88 45.19,46.48 45.19,81.81 46.87,83.5 P3.28
IO8  (via drill 0.3)
  Top 0.254: R53.1 25.4,117.66 27,117.66 v31.59,113.07 v31.6,113.07 | v21.44,52.17 20.98,51.7 20.98,43.73 21.25,43.46 21.25,43.02 U1.12
  Bottom 0.254: v31.6,113.07 31.73,112.94 31.73,112.71 20.98,101.96 20.98,52.63 v21.44,52.17
IO9
  Top 0.254: U1.17 25.31,47.07 40.21,47.07 41.53,48.39 41.53,83.06 46.97,88.5 P3.38
IO10  (via drill 0.3)
  Top 0.254: P3.21 48.61,80 48.39,79.78 v47.6,79.78 | U1.18 39.54,48.33 40.92,49.71 v40.92,79.78
  Bottom 0.254: v47.6,79.78 v40.92,79.78
IO11/MIDI_OUT
  Top 0.406: 31.15,49.59 R7.1
  Top 0.813: U1.19 31.15,49.59
IO12/MIDI_IN
  Top 0.406: U1.20 38.98,50.87 40.23,52.12 40.23,89.2 44.65,93.62 44.65,94.28 | U7.4 44.65,94.28 | R9.2 44.68,94.26 44.65,94.28
IO13  (via drill 0.3)
  Top 0.254: P3.20 48.89,79.5 48.56,79.17 v48,79.17 | U1.21 25.31,52.15 38.51,52.15 39.55,53.19 v39.55,79.17
  Bottom 0.254: v48,79.17 v39.55,79.17
IO14  (via drill 0.3)
  Top 0.254: P3.23 57.01,81 v47.8,81 | U1.22 37.84,53.41 38.93,54.5 v38.93,81
  Bottom 0.254: v47.8,81 v38.93,81
IO15
  Top 0.254: U1.8 16.43,41.43 17.45,40.41 38.3,40.41 44.6,46.71 44.6,82.07 46.53,84 P3.29
IO16
  Top 0.254: U1.9 17.7,42.09 18.82,40.97 37.97,40.97 44.02,47.02 44.02,82.35 46.17,84.5 P3.30
IO17/I2C_SDA  (via drill 0.3)
  Top 0.406: P4.5 v56.99,16 52.02,16 49.52,18.5 P1.5 22.89,18.49 v21.77,17.37 21.22,16.83 I2C.2 | v56.16,34.42 56.16,33.44 R47.1 | v19.15,41.76 19.15,42.57 U1.10
  Bottom 0.406: v56.99,16 56.99,33.59 v56.16,34.42 | v19.15,41.76 19.15,19.99 v21.77,17.37
IO18/I2C_SCL  (via drill 0.3)  (1 unrouted)
  Top 0.406: P4.4 51.37,15 48.87,17.5 P1.4 24.36,17.5 24.08,17.22 v24,17.14 23.22,16.36 I2C.1 | R42.1 51.57,31.93 R27.1 v48.72,31.93 | v20.04,41.76 20.04,42.55 U1.11
  Bottom 0.406: v48.72,17.5 v48.72,31.93 | v20.04,41.76 20.04,21.11 v24,17.14
IO19  (via drill 0.3)
  Top 0.305: 92.25,153.75 R20.2 | U1.13
  Top 0.406: 92.25,153.75 92.25,149.17 62.05,118.97 v31.39,118.97 | v22.99,43.74 22.99,42.96 U1.13
  Bottom 0.406: v22.99,43.74 22.99,47.68 18.39,52.27 18.39,117.88 19.48,118.97 v31.39,118.97 | v31.39,118.97 | v31.39,118.97
IO20  (via drill 0.3)
  Top 0.305: U1.14
  Top 0.406: v93.07,150.14 93.07,148.59 62.69,118.21 v31.39,118.21 | v91.44,150.14 91.44,153.03 R21.2 | v23.82,43.74 23.82,42.98 U1.14
  Bottom 0.254: v31.39,118.21 31.41,118.21 v31.38,118.21 v31.38,118.2
  Bottom 0.406: v93.07,150.14 v91.44,150.14 | v23.82,43.74 23.82,48.18 19.15,52.86 19.15,117.42 19.94,118.21 25.78,118.21 | 25.78,118.21 v31.39,118.21 | v31.38,118.2 31.35,118.2 31.35,118.21 | 31.35,118.21 31.36,118.21 | 31.35,118.21 31.32,118.21 31.32,118.2 25.78,118.2 | 25.78,118.21 25.78,118.2 | 25.78,118.2 25.77,118.2 25.77,118.21
IO21  (via drill 0.3)
  Top 0.254: P3.22 48.22,80.5 v48.12,80.4 | v38.33,80.4 38.33,55.17 37.85,54.69 25.31,54.69 U1.23
  Bottom 0.254: v38.33,80.4 v48.12,80.4
IO38  (via drill 0.3)
  Top 0.254: P3.36 47.57,87.5 42.77,82.7 v42.77,61.7 | U1.31 18.97,61.13 19.53,61.7 v25.83,61.7
  Bottom 0.254: v25.83,61.7 v42.77,61.7
IO39  (via drill 0.3)
  Top 0.254: R40.1 P3.40 v61.7,89.5
  Top 0.305: U1.32 17.7,66.39 20.52,69.22 v22,69.22
  Bottom 0.254: v22,69.22 52.22,69.22 61.7,78.69 v61.7,89.5
IO40  (via drill 0.3)
  Top 0.254: P3.42 59.46,90.5 59.79,90.83 v60.94,90.83
  Top 0.305: U1.33 16.43,66.24 20.12,69.93 v22.5,69.93
  Bottom 0.254: v22.5,69.93 51.84,69.93 60.94,79.02 v60.94,90.83
IO41  (via drill 0.3)
  Top 0.254: R45.1 54.35,90 P3.41 60.12,90 v60.27,90.15
  Top 0.305: U1.34 15.16,66.09 19.74,70.66 v22,70.66
  Bottom 0.254: v22,70.66 51.51,70.66 60.27,79.43 v60.27,90.15
IO42
  Top 0.305: 13.89,66 U1.35 13.89,69.44 FB1.2
IO45  (via drill 0.3)
  Top 0.254: P3.19 57.03,78.99 49.15,78.99 47.5,77.34 v47.5,58.7
  Top 0.305: v26.3,58.7 25.52,58.7 U1.26
  Top 0.406: U1.26 24.2,58.48 22.45,56.74 v14.58,56.74 | v11.02,39.19 R4.2
  Bottom 0.254: v26.3,58.7 v47.5,58.7
  Bottom 0.406: v11.02,39.19 11.02,50.11 14.58,53.67 v14.58,56.74
IO46
  Top 0.254: U1.16 39.82,45.78 42.14,48.11 42.14,82.83 47.31,88 P3.37
IO47  (via drill 0.3)
  Top 0.406: v15.24,55.93 25.29,55.93 U1.24 | R59.2 15.24,148.97 v15.24,149.56
  Bottom 0.406: v15.24,55.93 v15.24,149.56
IO48  (via drill 0.3)
  Top 0.406: v67.13,33.73 R41.2 | v26.3,57.2 26.29,57.22 U1.25
  Bottom 0.406: v26.3,57.2 61.37,57.2 64.64,53.92 64.64,36.22 v67.13,33.73
LCD_RST
  Top 0.254: P3.7 C15.2 R1.1
LED+  (via drill 0.3)
  Top 0.254: P3.49 P3.50 55.98,94.26 56.97,94.23
  Top 0.406: v58.9,125.8 19.11,125.8 17.71,127.19 | C12.2 14.75,132.23 D1.- C11.2 v16.61,128.29 17.71,127.19 | U2.5 15.85,139.55 16.05,139.75 v16.61,139.75 | R46.1 17.71,127.24 17.71,127.19
  Top 0.61: v58.9,94.25 56.97,94.25 56.97,94.23
  Bottom 0.406: v58.9,94.25 v58.9,125.8 | v16.61,128.29 v16.61,139.75
LED-  (via drill 0.3)
  Top 0.254: P3.47 P3.48 56.42,93.5 56.19,93.27
  Top 0.406: U2.3 16.8,133.46 R32.2 R33.2 16.74,131.93 16.74,130.32 17.79,129.27 | 17.79,129.27 17.8,129.27 17.8,129.3 R46.2 | 17.79,129.27 17.88,129.37 18.33,129.37 21.21,126.49 v59.61,126.49 arc90 v59.61,126.5
  Top 0.61: v59.61,93.27 56.19,93.27
  Bottom 0.406: v59.61,93.27 v59.61,126.5
LOUT  (via drill 0.3)
  Top 1.016: AUDIO_CONN1.2 38.42,149.2 AUDIO_CONN1.4 38.57,133.18 v38.58,133.17 | R68.1 23.9,103.83 v23.9,103.07 23.9,102.17 C84.1
  Bottom 1.016: v38.58,133.17 38.58,117.75 v23.9,103.07
LRC
  Top 0.305: U11.15 22.22,119.32 R54.2
N$1
  Top 0.61: D6.1 C47.2 R11.1
N$2
  Top 0.406: R26.1 16.2,86.16 16.2,87.13 Q4.1
N$3
  Top 0.406: Q3.1 17.36,80.91 18.77,82.32 R25.1
N$4
  Top 0.61: R52.1 R50.2 R49.1 C61.1
N$5
  Top 0.254: P3.4 54.58,71.5 R66.2 R65.1
N$6
  Top 0.254: USB-KEY.A5 91.83,157.29 R15.2
N$7
  Top 0.406: PWR.C R19.2
N$8
  Top 0.61: C48.2 D6.3
N$9
  Top 0.61: U4.1 59.75,36.41 59.46,36.7 59.46,41.02 | 59.46,41.02 59.46,41.81 L2.P$2 | 59.46,41.02 59.51,41.07 C48.1 C49.2 66.75,41.07 D9.+
N$10
  Top 0.254: USB-TTL.A5 21.94,155.74 R13.2
N$11
  Top 0.254: USB-TTL.B5 18.94,155.82 R12.2
N$12
  Top 0.61: C49.1 65.86,42.81 D7.3
N$13
  Top 0.61: R18.2 C50.2 D7.2
N$14
  Top 0.254: R14.2 89.2,157.13 88.84,157.5 88.84,158.43 USB-KEY.B5
N$15
  Top 0.61: U4.3 63.06,38.31 R52.2
N$16
  Top 0.61: R30.2 R3.1 74.64,36.78 RW1.2 77.13,36.54 RW1.3
N$17
  Top 0.406: L1.P$2 14.61,136.3 U2.1 14.88,136 D1.+ 14.4,134.01 R23.2
  pour Top: 8.59,135.23 12.32,135.23 12.85,134.7 12.85,133.68 15.11,133.68 15.11,136.8 8.59,136.8
N$18
  Top 0.406: R35.1 59.94,33.4 Q1.3
N$19
  Top 0.61: U4.4 56.29,38.31 R64.1
N$20
  Top 0.406: Q1.1 64.51,31.38 R43.2 R41.1
N$21
  Top 0.584: USB-TTL.VBUS1 23.13,158.92 22.65,159.4 22.65,160.16 | USB-TTL.VBUS2 18.24,158.93 18.59,159.27 18.59,159.54 18.58,159.55 18.58,160.22 19.32,160.97 27.03,160.97 FB2.1
  Top 0.61: 22.65,160.16 22.65,160.81 | 22.65,160.81 22.68,160.84 | 19.32,160.97 22.5,160.97 22.65,160.81
N$22
  Top 0.406: C2.2 R23.1
N$23  (via drill 0.3)
  Top 0.813: R5.2 v53.03,108.15 | MIDI_IN_CONN2.3 55.65,142.61 v53.03,140
  Top 1.016: MIDI_IN_CONN2.3 MIDI_IN_CONN2.5
  Bottom 0.813: v53.03,108.15 v53.03,140
N$24
  Top 0.406: U2.4 17.3,139.11 17.3,140.08 16.59,140.79 R39.1 R31.2 16.46,143.26 Q7.3
N$25
  Top 0.406: L3.P$2 5.96,127.13 6.1,127
  Top 0.61: L3.P$2 6.23,126.77 7.59,126.77 8.52,125.85 U9.1 12.46,123.65 D12.A
N$26
  Top 0.813: R5.1 D4.- 49.73,107.35 U7.1
N$27  (via drill 0.3)
  Top 0.813: v54.71,94.26 R6.2 | MIDI_OUT_CONN3.3 68.98,140.53 68.99,140.53 68.99,138.71 61.08,130.8 v54.71,130.8
  Top 1.016: MIDI_OUT_CONN3.3 MIDI_OUT_CONN3.5
  Bottom 0.813: v54.71,94.26 v54.71,130.8
N$28  (via drill 0.3)
  Top 0.61: C69.2 7.39,116 | 7.39,116 7.39,116.69 | 7.39,116.69 7.37,116.71 | R69.2 6.04,116.03 | 7.26,116.03 7.37,116.03 7.39,116 | 7.39,116.69 7.39,116.71 R48.1 7.42,116.18 7.26,116.03 | 7.26,116.03 6.04,116.03 | 6.04,116.03 6.02,116.05 v6.02,117.3 | v6.02,122.53 6.62,123.13 U9.3
  Bottom 0.61: v6.02,117.3 v6.02,122.53
N$29
  Top 0.406: Q7.1 16.85,147.33 R60.2 R59.1
N$30
  Top 0.406: U6.2 20.07,147.4 R28.1
N$31
  Top 0.406: R61.2 8.52,119.79 U9.6
N$32
  Top 0.406: 7.59,121.25 U9.5 7.57,119.15 | 7.57,119.15 7.57,118.36 7.47,118.26 R62.1 | R56.1 7.47,119.25 7.57,119.15
N$33
  Top 0.711: U8.4 C66.1 | C66.1 78.47,47.48 | C66.1
N$35  (via drill 0.3)
  Top 0.406: 32.64,49.63 R7.2
  Top 0.813: v37.41,82 v37.41,55.57 | R7.2 v37.41,49.58 | MIDI_OUT_CONN3.4 66.23,140.25 58.95,132.97 v50.04,132.97
  Top 1.016: MIDI_OUT_CONN3.2 66.08,149.2 MIDI_OUT_CONN3.4
  Bottom 0.813: v37.41,55.57 v37.41,49.58 | v37.41,82 50.04,94.62 v50.04,132.97
N$36  (via drill 0.3)
  Top 0.406: D4.+
  Top 0.813: 51.92,149.99 51.92,148.39 51.46,147.93 | U7.2 47.19,107.45 D4.+ 47.21,108.25 47.93,108.97 v51.46,108.97 | v51.46,142 51.46,147.93 | 51.46,147.93 51.46,150.64 51.05,151.05
  Top 1.016: MIDI_IN_CONN2.2 48.8,153.3 51.05,151.05 MIDI_IN_CONN2.4
  Bottom 0.813: v51.46,108.97 v51.46,142
N$43
  Top 0.305: U11.18 20.27,117.82 C73.1
  Top 1.016: C73.1 20.53,122.18 C79.+
N$44
  Top 0.305: U11.7 22.87,107.99 23.52,107.34 24.55,107.34 R67.2
N$45
  Top 0.305: U11.4 20.92,110.63 21.69,111.4 26.93,111.4 C77.1
N$46
  Top 0.406: U3.9 7.38,152.34 R17.2
N$47
  Top 0.305: U11.2 19.62,110.58 21.13,112.09 25.17,112.09 26.52,113.44 27.07,113.44 C77.2
N$49
  Top 0.406: U3.8 R2.2
N$76
  Top 0.61: U5.4 11.24,146.42 C45.1
OUTL
  Top 0.305: U11.6 22.22,107.51 R68.2
RESET  (via drill 0.3)
  Top 0.406: v10.08,44.15 U1.3 | RST.2 4.08,88.39 C8.1 12.25,88.39 Q4.3 13.89,88.36 v13.89,86.82 13.89,86.36 R16.1
  Bottom 0.406: v10.08,44.15 10.08,50.29 13.89,54.1 v13.89,86.82
ROUT  (via drill 0.3)
  Top 0.406: R67.1
  Top 1.016: AUDIO_CONN1.5 AUDIO_CONN1.3 42.55,159.47 v42.55,133.22 | C83.1 v26.36,99.47 25.81,100.03 25.81,100.64 | R67.1 25.81,100.64 | 24.79,99.54 24.79,99.62 25.81,100.64
  Bottom 1.016: v42.55,133.22 42.55,115.65 v26.36,99.47
RTS  (via drill 0.3)
  Top 0.406: v9.3,155.96 9.29,155.95 U3.6 | R25.2 18.77,87.37 16.98,89.17 16.82,89.33 | 16.82,89.33 Q4.2 | v13.89,89.75 16.4,89.75 16.82,89.33
  Bottom 0.406: v13.89,89.75 13.89,146.74 9.3,151.33 v9.3,155.96
RXD/IO44  (via drill 0.3)
  Top 0.406: v4.32,153.34 R2.1 | U1.36 12.62,61.34 v12.04,61.92
  Bottom 0.406: v12.04,61.92 12.04,145.62 v4.32,153.34
TP_INT  (via drill 0.3)
  Top 0.406: P4.2 v56.19,13 50.42,13 47.92,15.5 P1.2 | R36.1 R37.1 v56.19,27.74
  Bottom 0.406: v56.19,27.74 v56.19,13
TP_RST  (via drill 0.3)
  Top 0.406: 58.34,14 P4.3 | R44.1 57.79,31.9 | 57.79,31.9 C13.2 | 57.79,31.9 v57.79,31.14 v57.78,31.14 | v57.78,13.99 58.34,13.99 58.34,14 | 57.79,31.9 57.79,33.38 R35.2 | 58.34,14 50.9,14 48.4,16.5 P1.3
  Bottom 0.406: v57.78,31.14 v57.78,13.99
TXD/IO43  (via drill 0.3)
  Top 0.406: v4.57,151.76 R17.1 | U1.37 v11.35,61.26 v11.35,61.27
  Bottom 0.406: v11.35,61.27 11.35,144.98 v4.57,151.76
USB_D+
  Top 0.254: USB-KEY.A6 90.83,157.3 | 90.83,157.3 90.83,155.38 R21.1 | USB-KEY.B6 89.83,157.56 90.04,157.35 90.5,157.35 | 90.5,157.35 90.78,157.35 90.83,157.3 | 90.83,156.97 90.83,157.02 90.5,157.35 | 90.5,157.35 90.83,157.68 90.83,157.71
USB_D-
  Top 0.254: R20.1 91.33,156.24 USB-KEY.B7 91.33,159.24 91.08,159.49 90.53,159.49 90.33,159.29 USB-KEY.A7
VBAT
  Top 0.406: BAT.+ 26.43,139.79 C44.1 | C44.1 C40.1 26.49,142.32 | 26.49,142.32 R34.2 26.49,143.94 U6.5 | Q6.3 26.47,142.34 26.49,142.32 | D11.+ 26.36,139.72 C44.1
  pour Top: 26.97,134.62 25.65,134.62 24,136.27 24,142.85 26.21,145.06 28.07,145.06 28.07,144.48 27.05,143.46 27.05,134.7
VBUS  (via drill 0.3)
  Top 0.254: 18.24,157.15 v18.21,157.12
  Top 0.406: D10.A 30.05,156.05 30.05,156.21 29.87,156.21 29.87,156.29
  Top 0.584: U6.8 28.06,149.32 28.06,150.38 | 28.06,150.38 28.06,153.65 | 28.06,153.65 FB2.2 28.26,158.23 C38.1 | 31.33,158.19 31.17,158.19 31.11,158.12 31.24,158.12 R58.1 C38.1 | C38.1 | C38.1 29.87,158.21 29.87,156.29 | C39.1 27.01,150.48 C36.2 27.04,150.38 28.06,150.38 | D2.A 19.92,142.94 v19.92,144.23 | v27.21,153.47 27.88,153.47 arc90 28.06,153.65 | v19.92,144.23 19.19,144.23 arc-90 C37.1 | Q6.1 22.34,143.72 arc90 U6.4 20.54,144.86 arc90 v19.92,144.23
  Top 0.61: v23.14,157.12 23.14,156.54 23.39,156.29 23.44,156.29 | 23.44,156.29 25.04,156.29 | C4.2 23.39,156.24 23.44,156.29 | C6.2 24.89,156.13 25.04,156.29 | 25.04,156.29 29.87,156.29 | v18.21,157.12 17.35,156.26 17.35,155.87 17.29,155.81 C7.2
  Bottom 0.305: v23.14,157.12 23.16,157.1 23.16,157.08
  Bottom 0.61: v18.21,157.12 v23.14,157.12
  Bottom 0.762: v19.92,144.23 21.31,145.63 21.31,150.05 24.73,153.47 v27.21,153.47
  pour Top: 22.58,142.93 18.97,142.93 18.97,144.75 18.97,145.11 21.51,145.11 22.58,144.04
  pour Top: 26.42,148.41 26.42,156.62 28.34,156.62 28.36,152.73 28.32,151.43 28.35,150.06 28.35,148.41
  pour Top: 25.69,156.45 25.69,156.95 27.36,158.61 31.88,158.61 31.88,156.83 31.39,156.35 25.76,156.35 25.7,156.4
VCOM  (via drill 0.3)
  Top 0.254: v74.88,71.98 74.88,87.76 70.64,92 P3.45 | P3.5 64.68,72 v64.69,71.98 | v75.45,44.11 75.45,43.19 74.92,42.65 VCOM.T | VCOM.T 74.87,42.6 | VCOM.T
  Top 0.61: R29.1 73,38.33 R3.2 74.64,38.3 RW1.1 C52.2 VCOM.T
  Bottom 0.254: v64.69,71.98 v74.88,71.98 74.88,44.69 v75.45,44.11
VGH
  Top 0.254: P3.10 65.56,74.5 68.68,71.37 VGH.T
  Top 0.61: R18.1 R24.2 C51.2 68.45,53.98 | 68.45,53.98 C56.2 C57.2 68.45,58.98 VGH.T | D8.C 68.47,53.96 68.45,53.98
VGL
  Top 0.254: P3.9 65.24,74 66.67,72.57 VGL.T
  Top 0.61: R11.2 C46.2 R10.2 66.65,53.92 | 66.65,53.92 66.65,55.52 C58.2 C59.2 66.7,59.11 VGL.T | D5.A 66.65,53.92
VNEG
  Top 0.305: U11.5 21.57,106.14 C78.1
VOUT  (via drill 0.3)
  Top 0.406: Q6.2 22.34,139.75 D11.- 22.37,138.89 | 22.37,138.89 22.37,137.58 D3.C | D2.C 22.33,138.84 22.37,138.89
  Top 0.813: 21.67,137.03 21.67,137.14 D2.C 20.52,138.28 v20.52,137.41 | SW1.2@1 SW1.2 v5.4,142.26 5.4,141.71 5.41,141.71 | v20.52,124.8 16.35,124.8 13.87,127.28 10.31,127.28 v10.29,127.31 | v5.42,141.67 5.41,141.68 5.41,141.71 | 5.41,141.72 5.41,142.24 5.4,142.23 5.4,141.73 5.41,141.72 | 5.41,141.72 5.41,141.71
  Bottom 0.813: v20.52,137.41 v20.52,124.8 | v5.4,142.26 5.4,132.19 v10.29,127.31
  pour Top: 18.87,136.53 22.73,136.53 22.73,141.6 21.89,141.6 21.89,140.74 21.16,140 18.87,140
VPWR  (via drill 0.3)
  Top 0.254: SW1.3 3.84,139.86 3.94,139.95
  Top 0.406: U2.6 14.9,139.95 | 14.9,139.95 14.9,140.76 R39.2 | L1.P$1 11.53,140 | 11.53,140 12.8,140 | 12.8,140 14.85,140 14.9,139.95 | C43.2 12.9,140.1 12.8,140 | U5.3 11.24,140.29 11.53,140 | U5.1 9.34,139.96 9.35,139.95 | C41.1 7.87,140.06 7.98,139.95 | R56.2 2.87,119.84 v2.87,120.29
  Top 0.61: SW1.3@1 1.43,139.95 3.94,139.95 6.66,139.95 | 6.66,139.95 VPWR.T | 6.66,139.95 7.98,139.95 9.35,139.95 10.62,139.95 L1.P$1 | R57.2 2.76,130.83 2.95,130.83 v3.05,130.83 5.36,130.83 L3.P$1
  Top 0.813: SW1.3 3.9,139.83 6.91,139.83 6.88,139.8 5.46,139.8 5.36,139.7 5.36,130.83
  Bottom 0.406: v2.87,120.29 2.87,130.83 v3.05,130.83
  pour Top: 15.16,138.07 15.16,141.22 14.15,141.22 13.46,141.91 13.46,142.85 11.02,142.85 11.02,141.4 10.82,141.2 9.86,141.2 9.63,141.43 9.55,141.5 9.55,142.85 7.39,142.85 7.39,141.81 6.38,140.79 0.56,140.79 0.56,139.85 0.56,139.8 0.56,139.78 13.46,139.78 14.17,139.06 14.17,138.1 14.17,138.07

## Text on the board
tPlace: CHRG | C36 | Audio Out | MIDI In | MIDI Out | Off | C41 | + | - | On | + | - | Battery | tulip.computer | Tulip Creative Computer v4r11 | GND | +3V3 | IO17/SDA | IO18/SCL
tNames: U4
tValues: Close
Measures: Units: Inches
